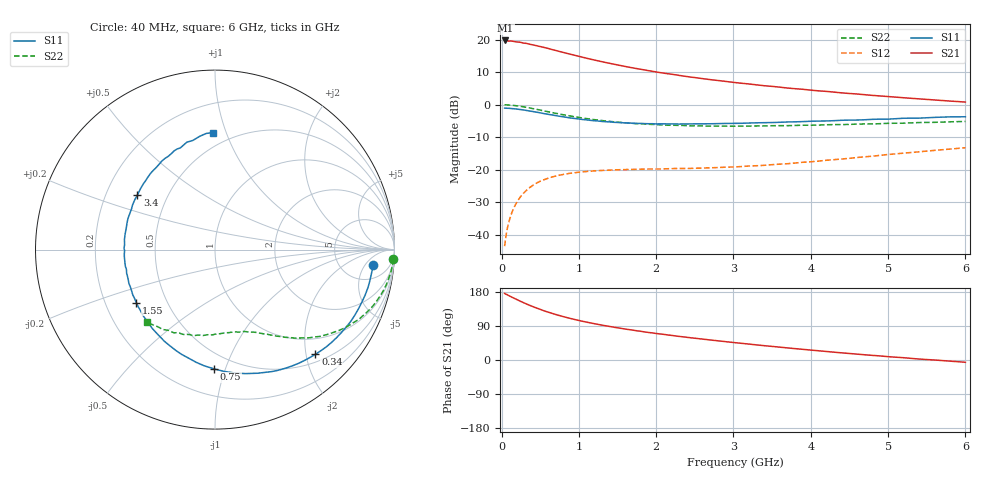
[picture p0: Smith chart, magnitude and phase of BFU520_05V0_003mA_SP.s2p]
! Filename:  P:\Prog\Test\Noise\ATS_data\Testdata_Net\03 Spar\BFU520_APG2013_37_A05_05p0V_003mA_SP_CM01_D.s2p
! Date/Time: Fri 26/Apr/2013 13:00:08
! BFU520_APG2013_37_A05_05p0V_1to20mA_SP_CM01_Bias3_R.s2p
! MDIF S-parameter v. bias file
! BFU520_APG2013_37_A05_05p0V_1to20mA_SP_CM01
! Date/time Tue Apr 23 15:26:19 2013
! VAR V_out= 5.0000
! VAR I_out= 2.9950
! VAR V_in= 0.8166
! VAR I_in= 0.0335
! Device data file deembeded for feedlines and parallel
! Original file: \03 Spar\BFU520_APG2013_37_A05_05p0V_003mA_SP_CM01_R.s2p
! Feed-files: PR047V01_250413_Feed1.s2p, PR047V01_250413_Feed2.s2p
! Parallel-file: PR047V01_250413_Par.s2p
# MHz S MA R 50
!  Freq-MHz  S11-mag  S11-arg  S21-mag  S21-arg  S12-mag  S12-arg  S22-mag  S22-arg
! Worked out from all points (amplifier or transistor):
!   98 points, 40 MHz to 6 GHz, reference 50 ohm
!   highest |S21| = 19.7 dB at 50 MHz (marker M1)
!   |S21| within 3 dB of that: start of sweep to 689.7 MHz
!   unconditionally stable (mu >= 1): 2.684 GHz to 4.776 GHz
!   at 300 MHz: K = 0.14, MSG = 22.8 dB, |S12| = -26.8 dB
!   at 1.6 GHz: K = 0.65, MSG = 15.8 dB, |S12| = -19.9 dB
!   at 6 GHz: K = 0.84, MSG = 7.0 dB, |S12| = -13.2 dB
!   S11 on the Smith chart (normalised r, x): 40 MHz: 10, -8; 340 MHz: 0.65, -2.18; 750 MHz: 0.38, -0.91; 1.55 GHz: 0.33, -0.27; 3.4 GHz: 0.34, +0.28; 6 GHz: 0.40, +0.90
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40  0.8857 -5.7  9.643 175.8  0.006726 86.0  0.9946 -3.0
50  0.8838 -7.1  9.669 174.1  0.008355 85.9  0.9956 -3.8
60  0.8823 -8.3  9.535 173.5  0.01005 84.9  0.9935 -4.7
70  0.881 -9.8  9.555 172.7  0.01167 84.2  0.9913 -5.4
120  0.8738 -17.0  9.492 167.3  0.0198 80.2  0.9815 -9.2
220  0.8487 -30.6  9.149 157.4  0.03495 72.3  0.9509 -16.5
340  0.8083 -46.2  8.613 146.4  0.05048 64.0  0.9004 -24.4
440  0.7716 -58.4  8.103 138.2  0.06119 58.0  0.8539 -30.0
550  0.7286 -71.0  7.555 129.8  0.07037 52.2  0.8007 -35.4
750  0.6639 -90.6  6.546 117.2  0.0827 44.2  0.7188 -43.1
900  0.6224 -103.7  5.907 109.2  0.08891 39.8  0.6673 -47.7
1050  0.5914 -115.3  5.338 102.1  0.09301 36.3  0.6232 -51.6
1300  0.5524 -131.9  4.564 92.0  0.09776 32.2  0.57 -56.7
1550  0.5286 -146.1  3.96 83.4  0.1005 29.7  0.5333 -61.1
1850  0.5114 -161.0  3.409 74.2  0.1026 28.2  0.5038 -66.0
2050  0.5079 -169.3  3.104 68.8  0.103 28.0  0.4893 -69.1
2500  0.5078 173.6  2.604 57.5  0.1057 29.1  0.4731 -76.0
3100  0.5176 153.9  2.132 44.1  0.1121 32.7  0.4684 -85.3
3400  0.5289 144.8  1.951 37.8  0.1172 34.5  0.4717 -90.1
4100  0.5599 127.7  1.629 24.4  0.136 38.3  0.4855 -101.4
5200  0.6187 104.7  1.276 6.0  0.1801 38.7  0.5193 -119.9
6000  0.652 91.1  1.096 -6.0  0.2181 35.1  0.5529 -133.6
